// TwinCAT 3 PLC project Untitled1
// ProgramVersion: 3.1.4022.2
// libraries:
//   Tc2_Drive, * (Beckhoff Automation GmbH)
//   Tc2_MC2, * (Beckhoff Automation GmbH)
//   Tc2_MC2_Drive, * (Beckhoff Automation GmbH)
//   Tc2_Standard, * (Beckhoff Automation GmbH)
//   Tc2_System, * (Beckhoff Automation GmbH)
//   Tc2_Utilities, * (Beckhoff Automation GmbH)
//   Tc3_Module, * (Beckhoff Automation GmbH)
//   VisuSymbols,3.5.10.0,System
// project tree:
//   DUTs/ Alm_AlarmHistoryType.TcDUT, Alm_AlarmType.TcDUT, Alm_AlmMsg.TcDUT, Alm_EventClass.TcDUT, manualstep.TcDUT, ST_AlarmID.TcDUT, ST_AlarmString.TcDUT, ST_Setting.TcDUT, ST_States.TcDUT
//   / GlobalTextList.TcGTLO, PlcTask.TcTTO, Visualization Manager.TcVMO
//   GVLs/ _01_Global_Variables.TcGVL
//   POUs/ Axis_IO.TcPOU, Axis_PTP_CoE.TcPOU, FB_Home_ByLimit.TcPOU, MAIN.TcPOU, ServoDriver_DI.TcPOU
//   VISUs/Visualizations/PH/ PH_JOGLINE.TcVIS
//   VISUs/Visualizations/ Visualization.TcVIS
// real-time tasks:
//   TASK PlcTask: cycle T#10ms, priority 20, ADS port 350
// motion (NC):
//   TASK NC-Task 1 SAF: cycle T#2ms, priority 4, ADS port 501
//   TASK NC-Task 1 SVB: cycle T#10ms, priority 8, ADS port 511
//   AXIS Axis 1 (id 1)
//     Dynamic: Acceleration=13453.5, Deceleration=13453.5, Jerk=40360.6
//     Velo: RefSearch=89.69024, RefSync=89.69024, SlowManual=448.4512, FastManual=2690.7072, Fast=8969.024, Maximum=8969.02
//     OtherSettings: AllowMotionCmdToSlave=true
//     encoder EncType=8
//       EncPara: ScaleFactorNumerator=104.8576, ScaleFactorDenominator=1048576, MaxCount=#xffffffff
//     drive DrvType=9
//       DrvPara: MaxCount=#xffffffff, DriveControlDWord=#x00030100
//         Analog: VeloReferenz=9865.9264, VeloScale=1.02400649589962, ScaleFactorActTorque=0.1
//         TimeComp: TaskDelayCycles=1
//     controller CtrType=1
//       CtrPara: PriorControlFactor=1
//         Observer: BandWidth=20
//   AXIS Axis 2 (id 2)
//     Dynamic: Acceleration=13453.5, Deceleration=13453.5, Jerk=40360.6
//     Velo: RefSearch=89.69024, RefSync=89.69024, SlowManual=448.4512, FastManual=2690.7072, Fast=8969.024, Maximum=8969.02
//     OtherSettings: AllowMotionCmdToSlave=true
//     encoder EncType=8
//       EncPara: ScaleFactorNumerator=104.8576, ScaleFactorDenominator=1048576, MaxCount=#x0036ee7f
//     drive DrvType=9
//       DrvPara: MaxCount=#xffffffff, DriveControlDWord=#x00030100
//         Analog: VeloReferenz=9865.9264, VeloScale=6, ScaleFactorActTorque=0.1
//         TimeComp: TaskDelayCycles=1
//     controller CtrType=1
//       CtrPara: PriorControlFactor=1
//         Observer: BandWidth=20
// I/O:
//   DEVICE Device 1 (EtherCAT), AmsNetId 169.254.43.76.2.1
//     Term 1 (EK1200) [EK1200-5000 EtherCAT Power supply (2A E-Bus)]
//       Term 2 (EL1008) [EL1008 8Ch. Dig. Input 24V, 3ms]
//       Term 3 (EL2004) [EL2004 4Ch. Dig. Output 24V, 0.5A]
//       Term 4 (EL1259) [EL1259 8Ch. Dig Input 24V/8Ch. Dig. Output 24V with Multi-Time-Stamp]
//       Term 5 (EL1004) [EL1004 4Ch. Dig. Input 24V, 3ms]
//       Term 6 (EL2024) [EL2024 4Ch. Dig. Output 24V, 2A]
//       Term 7 (EL3204) [EL3204 4Ch. Ana. Input PT100 (RTD)]
//       Term 8 (EK1521) [EK1521 1 port EtherCAT junction (FX-MultiMode)]
//       Term 9 (EL6601) [EL6601 1 Port Switch (Ethernet, CoE)]
//       Term 10 (EL6731-0010) [EL6731-0010 PROFIBUS DP Slave]
//       Term 11 (EK1110) [EK1110 EtherCAT extension]
//     Term 12 (EK1100) [EK1100 EtherCAT Coupler (2A E-Bus)]
//       Term 13 (EL1004) [EL1004 4Ch. Dig. Input 24V, 3ms]
//       Term 14 (EL2004) [EL2004 4Ch. Dig. Output 24V, 0.5A]
//       Term 15 (EL6900) [EL6900, TwinSAFE PLC]
//       Term 16 (EL2904) [EL2904, 4 Ch. Safety Output 24V, 0.5A, TwinSAFE]
//         modules: Module 1 (FSOES), Module 2 (DO)
//       Term 17 (EL1904) [EL1904, 4 Ch. Safety Input 24V, TwinSAFE]
//         modules: Module 1 (FSOES)
//       Term 18 (EK1110) [EK1110 EtherCAT extension]
//     Drive 19 (AX5206-0000-0210) [AX5206-0000-0210 EtherCAT Drive (SoE, 2 Ch.)]
// variable links:
//   NC-Task 1 SAF/Axes/Axis 1 <-> Device 1 (EtherCAT)/Drive 19 (AX5206-0000-0210)
//     Drive/Inputs/In/nDataIn1 <-> AT 1/Following distance
//     Drive/Inputs/In/nDcOutputTime <-> InfoData/DcOutputShift
//     Drive/Inputs/In/nState1 <-> AT 1/Drive status word @bit 8
//     Drive/Inputs/In/nState2 <-> AT 1/Drive status word
//     Drive/Inputs/In/nState4 @bit 1 <-> WcState/InputToggle
//     Drive/Inputs/In/nState4 <-> WcState/WcState
//     Drive/Outputs/Out/nCtrl1 <-> MDT 1/Master control word @bit 8
//     Drive/Outputs/Out/nDataOut1 <-> MDT 1/Position command value
//     Enc/Inputs/In/nDataIn1 <-> AT 1/Position feedback 1 value
//     Enc/Inputs/In/nDcInputTime <-> InfoData/DcInputShift
//     Enc/Inputs/In/nState4 @bit 1 <-> WcState/InputToggle
//     Enc/Inputs/In/nState4 <-> WcState/WcState
//   NC-Task 1 SAF/Axes/Axis 2 <-> Device 1 (EtherCAT)/Drive 19 (AX5206-0000-0210)
//     Drive/Inputs/In/nDataIn1 <-> AT 2/Following distance
//     Drive/Inputs/In/nDcOutputTime <-> InfoData/DcOutputShift
//     Drive/Inputs/In/nState1 <-> AT 2/Drive status word @bit 8
//     Drive/Inputs/In/nState2 <-> AT 2/Drive status word
//     Drive/Inputs/In/nState4 @bit 1 <-> WcState/InputToggle
//     Drive/Inputs/In/nState4 <-> WcState/WcState
//     Drive/Outputs/Out/nCtrl1 <-> MDT 2/Master control word @bit 8
//     Drive/Outputs/Out/nDataOut1 <-> MDT 2/Position command value
//     Enc/Inputs/In/nDataIn1 <-> AT 2/Position feedback 1 value
//     Enc/Inputs/In/nDcInputTime <-> InfoData/DcInputShift
//     Enc/Inputs/In/nState4 @bit 1 <-> WcState/InputToggle
//     Enc/Inputs/In/nState4 <-> WcState/WcState
//   Untitled1/Untitled1 Instance <-> Device 1 (EtherCAT)/Drive 19 (AX5206-0000-0210)
//     PlcTask Inputs/MAIN.axis1.IO.DriverDI.ErrorCode <-> AT 1/Diagnostic number
//   Untitled1/Untitled1 Instance <-> Device 1 (EtherCAT)/Term 1 (EK1200)/Term 2 (EL1008)
//     PlcTask Inputs/MAIN.axis1.IO.DriverDI.EL1008 <-> Channel 1/Input
//     PlcTask Inputs/MAIN.axis1.IO.DriverDI.EL1008 @bit 1 <-> Channel 2/Input
//     PlcTask Inputs/MAIN.axis1.IO.DriverDI.EL1008 @bit 3 <-> Channel 4/Input
//     PlcTask Inputs/MAIN.axis1.IO.DriverDI.EL1008 @bit 4 <-> Channel 5/Input
//     PlcTask Inputs/MAIN.axis1.IO.DriverDI.EL1008 @bit 5 <-> Channel 6/Input
//     PlcTask Inputs/MAIN.axis1.IO.DriverDI.EL1008 @bit 6 <-> Channel 7/Input
//     PlcTask Inputs/MAIN.axis1.IO.DriverDI.EL1008 @bit 7 <-> Channel 8/Input
//     PlcTask Inputs/MAIN.home_exe <-> Channel 3/Input
//   Untitled1/Untitled1 Instance <-> Device 1 (EtherCAT)/Term 1 (EK1200)/Term 5 (EL1004)
//     PlcTask Inputs/MAIN.axis1.IO.DriverDI.EL1004 <-> Channel 1/Input
//   Untitled1/Untitled1 Instance <-> NC-Task 1 SAF/Axes/Axis 1
//     PlcTask Inputs/MAIN.axis1.Ref.NcToPlc <-> Outputs/ToPlc
//     PlcTask Outputs/MAIN.axis1.Ref.PlcToNc <-> Inputs/FromPlc

CONFIGURATION Untitled1
    RESOURCE PLC ON TwinCAT3
        TASK PlcTask(INTERVAL := T#10ms, PRIORITY := 20);
        PROGRAM MAIN WITH PlcTask : MAIN;
    END_RESOURCE
END_CONFIGURATION

// ---- DUTs/Alm_AlarmHistoryType.TcDUT
TYPE Alm_AlarmHistoryType :
STRUCT
  	EventMessage:            	WSTRING;
	EventId:					INT;
   	EventTime:               	DT;
END_STRUCT
END_TYPE

// ---- DUTs/Alm_AlarmType.TcDUT
TYPE Alm_AlarmType :
STRUCT
      (*InPut*)
	EventId:					INT;
    EventMessage:			WSTRING;
    EventTime:                                 DT;
	EventActive:				BOOL;
	QuitRequired:				BOOL;
	QuitEvent:				BOOL;
	EventClass:				Alm_EventClass;
	AlarmMsg:				Alm_AlmMsg;
	AlarmlampOn:			BOOL;(*报警灯*)
	AutoRunOff:				BOOL;(*退出自动循环*)

	(* event actions OutPut	*)
	AlarmAction1:				BOOL;
	AlarmAction2:				BOOL;
	AlarmAction3:				BOOL;
	AlarmAction4:				BOOL;
	AlarmAction5:				BOOL;
	AlarmAction6:				BOOL;
	AlarmAction7:				BOOL;
	AlarmAction8:				BOOL;

       (*OutPut*)
	EventAlive:					BOOL;
    ShowlampOn:           		BOOL;
	InUse:                		BOOL;
END_STRUCT
END_TYPE;

// ---- DUTs/Alm_AlmMsg.TcDUT
TYPE Alm_AlmMsg :
STRUCT
	CN:		WSTRING:="中文";
	EN:		STRING:='En';	
END_STRUCT
END_TYPE

// ---- DUTs/Alm_EventClass.TcDUT
TYPE Alm_EventClass :
(
    NoAlarm                  :=0,(*无警报*)
    Message_1      :=1,(*信息*)
    Event_2            :=2,(*事件*)
    non_3                        :=3,(*暂无*)
    non_4                       :=4,(*暂无*)
    non_5                         :=5,(*暂无*)
    Alarm_6          :=6,(*不停机警报*)
    Stop_7                :=7(*停机警报*)
);
END_TYPE

// ---- DUTs/manualstep.TcDUT

TYPE manualstep :
(
	moveoff:=0,
    jogB,
	jogF,
	homing ,
	MoveRel,
	MoveABS,
	MoveVel,
	stop
);
END_TYPE

// ---- DUTs/ST_AlarmID.TcDUT
TYPE ST_AlarmID :
(*报警的id号，swen*)
STRUCT
	(*系统*)
	EtherCATBusErr:					INT:=1;(*EtherCAT总线错误*)
	SystemLoading:					INT:=2;(*系统启动中*)
	EmergentStop:					INT:=3;(*急停按钮*)
	ProductChangeNeedSave:			INT:=4;
	ProductLoadingNoPowerOff:		INT:=5;
	AirPressLow:					INT:=6;(*气压低!*)
	Prushing:						INT:=7;(*暂停中*)
	NeedHoming:						INT:=8;(*开机前请先找原点*)
	IsHoming:						INT:=9;(*正在找原点*)
	AutoStoping:					INT:=10;(*自动停机中*)
	AutoStopImediery:				INT:=11;(*马上停机中*)
	AutoRuning:						INT:=12;(*设备运行中*)
	ComErrorVS:						INT:=13;(*视觉控制器通讯异常*)
	ServoError:						INT:=14;(*伺服出错*)
	ServoHwError:					INT:=15;(*伺服驱动器报错，硬件报错*)
	ServoLimit:						INT:=16;(*伺服驱动器限位到*)
	CycleTimeOut:					INT:=17;(*循环时间超时*)
	ModbusRtuError:					INT:=18;(*ModbusRtu总线错误*)
	RobotError1:					INT:=19;(*机器人错误*)
	RobotError2:					INT:=20;(*机器人错误*)
	StepServoError:					INT:=21;(*步进驱动器报错*)
	RobotSN_Error:					INT:=22;(*机器人序列号异常*)

	(*程序逻辑*)
	ClampVacuum:					INT:=26;(*机器人1真空吸取失败*)








	(*序列号*)
	Machime_SoftHwDif:				INT:=50;(*软硬件不匹配*)
	Machime_Alarm_NeedKey:			INT:=51;(*系统即将进入维护模式*)
	Machime_Stop_NeedKey:			INT:=52;(*系统已经进入维护模式*)

END_STRUCT
END_TYPE

// ---- DUTs/ST_AlarmString.TcDUT
TYPE ST_AlarmString :
STRUCT
	chinese:		STRING:='CN';
	english:		STRING:='EN';
END_STRUCT
END_TYPE

// ---- DUTs/ST_Setting.TcDUT
TYPE ST_Setting :
STRUCT
	(*系统*)
	gcSimulationMode:		BOOL;
	JogVelocity:			REAL:=20;
	AutoVelocity:			REAL:=500;(*皮带的速度*)
	ClampVelocity:			REAL:=2000;(*机械手的速度*)

	tCutTime:				REAL:=0.5;(*剪断时间*)

	ZPickUpHeight:			REAL:=200;(*抓起来的高度*)
	XPlacePos:				REAL:=450;(*抓过去的X距离*)
	YPlacePos:				REAL:=330;(*抓过去的Y距离*)
	ZPlacePos:				REAL:=-650;(*放到地板的高度*)
	Box_Longth:				REAL:=215;(*箱子长*)
	Box_Width:				REAL:=190;(*箱子宽*)
	Box_Height:				REAL:=198;(*箱子高*)

END_STRUCT
END_TYPE

// ---- DUTs/ST_States.TcDUT
TYPE ST_States :
STRUCT
	ManualModeIsActive:				BOOL;(*手动模式*)
	AutoModeIsActive:				BOOL;(*自动模式*)
	MachineRunInCycle:				BOOL;(*自动运行中*)
	GoPauseState:					BOOL;(*请求暂停记忆*)
	AutoStoping:					BOOL;(*自动停机中*)
	ResetAlarm:						BOOL;(*报警复位*)
	GoHome:							BOOL;(*请求找原点*)


	(*电机*)
	HomeDone:						BOOL;(*原点完成*)
	Motor_PowerOn:				BOOL;(*上电完成*)
	Motor_HomeDone:				BOOL;(*原点完成*)
	Motor_SwError:				BOOL;(*电机NC软件出错*)
	Motor_SwErrId:				UDINT;
	Motor_Limit:				BOOL;(*电机限位*)
	Motor_HwError:				BOOL;(*电机硬件出错*)

	Hmi_btHome:						BOOL;(*画面按钮*)(*回原点*)
	Hmi_btAutoRun:					BOOL;(*画面按钮*)(*开始*)
	Hmi_btAutoStop:					BOOL;(*画面按钮*)(*停止*)
	Hmi_btPause:					BOOL;(*画面按钮*)(*暂停*)


	(*状态*)
	ConvCanRun:						BOOL:=TRUE;(*传送带启动允许*)

	ActBoxId:						INT;(*当前进箱子的ID号*)


END_STRUCT
END_TYPE

// ---- GVLs/_01_Global_Variables.TcGVL
{attribute 'Tc2GvlVarNames'}
VAR_GLOBAL
	DATA:						ST_States;	(*状态*)
END_VAR

// ---- POUs/MAIN.TcPOU
PROGRAM MAIN
VAR
	axis1: Axis_PTP_CoE;	
    home_exe AT%I*:BOOL;
    mstep:manualstep;
	AutoMode: BOOL;
END_VAR

axis1.sName:="X轴";
axis1.areset( );                                //刷新IO，读取轴状态、复位
axis1.aPower( );                                //使能

IF axis1.Ref.Status.ControlLoopClosed AND NOT AutoMode THEN      //判断使能成功，调用手动模式下点动指令
axis1.aManualJOG(Velo:=100 ,);
END_IF


IF home_exe THEN axis1.aHome(execute:=TRUE);  
	ELSE axis1.aHome(execute:=FALSE);
END_IF

IF automode THEN                              //自动模式下的指令使用
logic();
END_IF

ACTION logic:
CASE mstep OF 
	moveoff:
	   axis1.aStop(execute:=FALSE);
	   axis1.aMoveOff();
	jogB:
	   axis1.aJogB(execute:=TRUE,velo:=100); 
	jogF:
	   axis1.aJogF(execute:=TRUE,velo:=100); 
    homing:  
       axis1.aHome(execute:=TRUE);
       IF axis1.done THEN
	    mstep:=moveoff;
       END_IF
	MoveRel:
	   axis1.aMoverel(execute:=TRUE,Target:=100,velo:=100);
	   IF axis1.done THEN
	    mstep:=moveoff;
	   END_IF
	Moveabs:
	   axis1.aMoveabs(execute:=TRUE,Target:=100,velo:=100);
	   IF axis1.done THEN
	    mstep:=moveoff;
	   END_IF
	MoveVel:
	   axis1.aMoveVel(execute:=TRUE,velo:=100);
    stop:
	   axis1.aStop(execute:=TRUE);
END_CASE
END_ACTION

END_PROGRAM

// ---- POUs/Axis_PTP_CoE.TcPOU
FUNCTION_BLOCK Axis_PTP_CoE
VAR_INPUT
	Execute:				BOOL;
	bReset:					BOOL;
	Ref:					AXIS_REF;
	IO:						Axis_IO;
	mcJog:					MC_Jog;
	mcHome:					FB_Home_ByLimit;
	mcMoveAbsolute:			MC_MoveAbsolute;
	mcMoveRelative:			MC_MoveRelative;
	mcMoveVelocity:			MC_MoveVelocity;
	mcSoEReset:				FB_SoEReset;
	mcPower:				MC_Power;
	mcReset:				MC_Reset;
	mcStop:					MC_Stop;

	Target					:	LREAL;
	Velo					: 	LREAL;
	Jerk					:	LREAL := 0.0;
	Acc						:	LREAL := 0.0;
	Dec						:	LREAL := 0.0;

	sName:					WSTRING:="轴";
END_VAR
VAR
	Done:					BOOL;(*功能块执行完成状态*)
	Busy: 					BOOL;(*功能块正在执行状态*)
	Active:					BOOL;
	CommandAborted:			BOOL;
	Error:					BOOL;
	ErrorID:				UDINT;
END_VAR

;

ACTION aHome:
(*
TYPE MC_HomingMode :
(
	MC_DefaultHoming,		(* default homing as defined in the SystemManager encoder parameters *)
	MC_AbsSwitch, 		(* not implemented - Absolute Switch homing plus Limit switches *)
	MC_LimitSwitch, 		(* not implemented - Homing against Limit switches *)
	MC_RefPulse, 		(* not implemented - Homing using encoder Reference Pulse "Zero Mark" *)
	MC_Direct, 		(* Static Homing forcing position from user reference *)
	MC_Absolute, 		(* not implemented - Static Homing forcing position from absolute encoder *)
	MC_Block, 		(* not implemented - Homing against hardware parts blocking movement *)
	MC_ForceCalibration, 	(* set the calibration flag without performing any motion or changing the position *)
	MC_ResetCalibration  	(* resets the calibration flag without performing any motion or changing the position *)
);
END_TYPE

*)


mcHome(
	Execute:= 			Execute,
	Position:= 			,
	HomingMode:= 		,
	PosLimit:=			IO.snLimitP,
	NegLimit:=			IO.snLimitN,
	bCalibrationCam:= 	IO.snHome,
	Axis:= 				Ref,
	Done=>				Done,
	Busy=> 			Busy,
	Active=> 		Active,
	CommandAborted=> CommandAborted,
	Error=> 		Error,
	ErrorID=> 		ErrorID
	);
END_ACTION

ACTION aIO:
IO.DriverDI();(*调用axis_io*)

IO.snLimitP	:=IO.DriverDI.bLimitSenser_P;
IO.snLimitN	:=IO.DriverDI.bLimitSenser_N;
IO.snHome	:=IO.DriverDI.bHomeSenser;


IF IO.snLimitP
OR IO.snLimitN THEN(*极限*)
	DATA.Motor_Limit:=TRUE;
END_IF

IF IO.DriverDI.bHwError THEN(*×硬件故障*)
	DATA.Motor_HwError:=TRUE;
END_IF

IF Ref.Status.Error THEN(*NC的故障状态*)
	DATA.Motor_SwError:=TRUE;
	DATA.Motor_SwErrId:=Ref.Status.ErrorID;
	
END_IF
END_ACTION

ACTION aJogB:
mcJog(
	JogForward:= 	FALSE,
	JogBackwards:= 	Execute,
	Mode:= 			MC_JOGMODE_CONTINOUS,
	Position:= 		,
	Velocity:= 		Velo,
	Acceleration:= 	Acc,
	Deceleration:= 	Dec,
	Jerk:= 			Jerk,
	Axis:= 			Ref,
	Busy=> 			Busy,
	Active=> 		Active,
	CommandAborted=> CommandAborted,
	Error=> 		Error,
	ErrorID=> 		ErrorID
	);
END_ACTION

ACTION aJogF:
mcJog(
	JogForward:= 	Execute,
	JogBackwards:= 	FALSE,
	Mode:= 			MC_JOGMODE_CONTINOUS,
	Position:= 		,
	Velocity:= 		Velo,
	Acceleration:= 	Acc,
	Deceleration:= 	Dec,
	Jerk:= 			Jerk,
	Axis:= 			Ref,
	Busy=> 			Busy,
	Active=> 		Active,
	CommandAborted=> CommandAborted,
	Error=> 		Error,
	ErrorID=> 		ErrorID
	);
END_ACTION

ACTION aManualJOG:
(*
TYPE E_JogMode :
(
	MC_JOGMODE_STANDARD_SLOW, (* motion with standard jog parameters for slow motion *)
	MC_JOGMODE_STANDARD_FAST, (* motion with standard jog parameters for fast motion *)
	MC_JOGMODE_CONTINOUS,     (* axis moves as long as the jog button is pressed using parameterized dynamics *)
	MC_JOGMODE_INCHING,       (* axis moves for a certain relative distance *)
	MC_JOGMODE_INCHING_MODULO (* axis moves for a certain relative distance - stop position is rounded to the distance value *)
);
END_TYPE

*)

mcJog(
	JogForward:= 	IO.btManualJogF,
	JogBackwards:= 	IO.btManualJogB,
	Mode:= 			MC_JOGMODE_CONTINOUS,
	Position:= 		,
	Velocity:= 		Velo,
	Acceleration:= 	Acc,
	Deceleration:= 	Dec,
	Jerk:= 			Jerk,
	Axis:= 			Ref,
	Busy=> 			Busy,
	Active=> 		Active,
	CommandAborted=> CommandAborted,
	Error=> 		Error,
	ErrorID=> 		ErrorID
	);
END_ACTION

ACTION aMoveAbs:
mcMoveAbsolute(
	Execute:= 		Execute,
	Position:= 		Target,
	Velocity:= 		Velo,
	Acceleration:= 	Acc,
	Deceleration:= 	Dec,
	Jerk:= 			Jerk,
	Axis:= 			Ref,
	Done=> 			Done,
	Busy=> 			Busy,
	Active=> 		Active,
	CommandAborted=> CommandAborted,
	Error=> 		Error,
	ErrorID=> 		ErrorID
	);
END_ACTION

ACTION aMoveOff:
(*触发条件复位*)
mcHome(
	Execute:= 		FALSE,
	Axis:= 			Ref,
	);

mcJog(
	JogForward:= 	FALSE,
	JogBackwards:= 	FALSE,
	Axis:= 			Ref,
	);

mcMoveAbsolute(
	Execute:= 		FALSE,
	Axis:= 			Ref,
	);

mcMoveRelative(
	Execute:= 		FALSE,
	Axis:= 			Ref,
	);

mcMoveVelocity(
	Execute:= 		FALSE,
	Axis:= 			Ref,
	);

Done:=FALSE;
Busy:=FALSE;
Active:=FALSE;
CommandAborted:=FALSE;
Error:=FALSE;
END_ACTION

ACTION aMoveRel:
mcMoveRelative(
	Execute:= 		Execute,
	Distance:= 		Target,
	Velocity:= 		Velo,
	Acceleration:= 	Acc,
	Deceleration:= 	Dec,
	Jerk:= 			Jerk,
	Axis:= 			Ref,
	Done=> 			Done,
	Busy=> 			Busy,
	Active=> 		Active,
	CommandAborted=> CommandAborted,
	Error=> 		Error,
	ErrorID=> 		ErrorID
	);
END_ACTION

ACTION aMoveVel:
mcMoveVelocity(
	Execute:= 		Execute,
	Direction:= 	,
	Velocity:= 		Velo,
	Acceleration:= 	Acc,
	Deceleration:= 	Dec,
	Jerk:= 			Jerk,
	Axis:= 			Ref,
	InVelocity=> 	Done,
	Busy=> 			Busy,
	Active=> 		Active,
	CommandAborted=> CommandAborted,
	Error=> 		Error,
	ErrorID=> 		ErrorID );
END_ACTION

ACTION aPower:
mcPower(
	Enable:= 			TRUE,
	Enable_Positive:= true	,
	Enable_Negative:=true 	,
	Override:= 		,
	BufferMode:= 	,
	Axis:= 			Ref,
	Status=> 		,
	Busy=> 			Busy,
	Active=> 		Active,
	Error=> 		Error,
	ErrorID=> 		ErrorID
	);
END_ACTION

ACTION aReset:
aIO();(*硬件IO刷新*)
Ref.ReadStatus();(*轴状态字刷新*)



(*NC复位*)
mcReset(
	Execute:= 	(bReset OR DATA.ResetAlarm)
				AND Ref.Status.Error,
	Axis:= 		Ref,
	);
(*AX5000驱动器复位*)
mcSoeReset(
	Execute:= 	(bReset OR DATA.ResetAlarm)
				AND Ref.Status.Error,
	Axis:= 		Ref,
	);


(*遇极限后禁止往极限方向运行*)
mcPower(
	Enable:= 			,
	Enable_Positive:= 	NOT IO.snLimitP
						
						AND mcPower.Enable,
	Enable_Negative:= 	NOT IO.snLimitN
					
						AND mcPower.Enable,
	Override:= 		,
	Axis:= 			Ref,

	);
END_ACTION

ACTION aStop:
aMoveOff(); (*触发条件复位*)
 
mcStop(
	Execute:= 		Execute,
	Deceleration:= 	Dec,
	Jerk:= 			Jerk,
	Options:= 		,
	Axis:= 			Ref,
	Done=> 			Done,
	Busy=> 			Busy,
	Active=> 		Active,
	CommandAborted=> CommandAborted,
	Error=> 		Error,
	ErrorID=> 		ErrorID
	);
END_ACTION

END_FUNCTION_BLOCK

// ---- POUs/Axis_IO.TcPOU
FUNCTION_BLOCK Axis_IO
VAR_INPUT
	snHome:			BOOL;(*原点*)
	snLimitP:		BOOL;(*正限*)
	snLimitN:		BOOL;(*负限*)
	btManualJogF:	BOOL;(*点动按钮正*)
	btManualJogB:	BOOL;(*点动按钮负*)
	DriverDI:		ServoDriver_DI;(*伺服驱动器的输入*)
END_VAR

;

END_FUNCTION_BLOCK

// ---- POUs/ServoDriver_DI.TcPOU
FUNCTION_BLOCK ServoDriver_DI(*伺服驱动器的数字量输入*)
VAR_INPUT

END_VAR
VAR_OUTPUT
END_VAR
VAR
	di_UDint AT%I*:			UDINT;(*数字量*)
	di_Uint AT%I*:			UINT;(*数字量*)
	ErrorCode AT%I*:		UDINT;(*伺服硬件错误号*)
	EL1008 AT%I*:           BYTE;
	EL1004 AT%I*:           BOOL;

	bHomeSenser:			BOOL;(*原点信号*)
	bLimitSenser_P:			BOOL;(*正向限位*)
	bLimitSenser_N:			BOOL;(*负向限位*)
	bHwError:					BOOL;(*硬件报警*)
END_VAR




	bHomeSenser 	:= di_UDint.2 OR di_Uint.2OR EL1004;	(*home=2, Plimit=1,Nlimit=0*)
	bLimitSenser_P 	:= di_UDint.1 OR di_Uint.4OR EL1008.0;
	bLimitSenser_N 	:= di_UDint.0 OR di_Uint.5OR EL1008.1;

IF errorcode=16#D012 OR errorcode=16#D013 THEN
	 bHwError			:= FALSE;
ELSE bHwError			:= TRUE; 
END_IF                                                       (* ErrorCode<>0;*)

END_FUNCTION_BLOCK

// ---- POUs/FB_Home_ByLimit.TcPOU
FUNCTION_BLOCK FB_Home_ByLimit
(*========================================
轴在任意位置回零功能块，无需考虑回零方向问题
默认回零方向：先负方向找原点,如果碰到负极限则改为正方向找原点

 By Swen & Richel	2017/2/8
==========================================*)
VAR_IN_OUT
	Axis				:	AXIS_REF;	(* B *)
END_VAR
VAR_INPUT
	Execute			:	BOOL;	(* B *)
	PosLimit		:BOOL;			(*正极限位信号*)
	NegLimit		:BOOL;			(*负极限位信号*)
	Position		:	LREAL			(* B *) := DEFAULT_HOME_POSITION;
	HomeingVelo		:LREAL	:=20;
	HomingMode		: 	MC_HomingMode;	(* V *)
	BufferMode		:	MC_BufferMode;		(* E *)
	Options			: 	ST_HomingOptions;	(* V *)	(* Beckhoff proprietary input *)
	bCalibrationCam 	: 	BOOL;	(* V *)	(* Beckhoff proprietary input *)


END_VAR
VAR_OUTPUT
	Done			:	BOOL;	(* B *)
	Busy			: 	BOOL;	(* E *)
	Active			: 	BOOL;	(* E *)
	CommandAborted	:	BOOL;	(* E *)
	Error			:	BOOL;	(* B *)
	ErrorID			:	UDINT;	(* E *)
END_VAR
VAR
	mcJog			:MC_Jog;
	mcHome			:MC_Home;
	HomeStep: INT;
END_VAR

IF  NOT Execute THEN
	mcJog.JogForward		:=FALSE;
	mcJog.JogBackwards		:=FALSE;
	mcHome.Execute			:=FALSE;
	done					:=FALSE;
	busy					:=FALSE;
	Error					:=FALSE;
	HomeStep				:=0;

END_IF


CASE HomeStep OF

0:
	busy	:=FALSE;
	Done	:=FALSE;
	IF 	Execute AND NOT Error  THEN

		IF	HomingMode  =MC_DefaultHoming  THEN  		 (*回零模式判断*)
			HomeStep	:=100;
		ELSE
			HomeStep	:=400;
		END_IF
		busy		:=TRUE;
		ErrorID		:=0;
	END_IF

100:
	mcJog.JogForward		:=FALSE;
	mcJog.JogBackwards		:=TRUE;		 (*先向负限位方向运动*)
	IF	NegLimit THEN
		mcJog.JogBackwards		:=FALSE;

		HomeStep	:=200;
	ELSIF  bCalibrationCam THEN
		mcJog.JogBackwards		:=FALSE;
		IF Axis.Status.NotMoving THEN
			HomeStep	:=400;
		END_IF
	ELSIF mcJog.Error THEN
			HomeStep	:=1000;

	END_IF

200:
	mcJog.JogBackwards		:=FALSE;
	mcJog.JogForward		:=TRUE;		(*向正限位方向运动*)

	IF	bCalibrationCam THEN
		HomeStep	:=300;
	ELSIF PosLimit THEN(*出错碰限位*)
		mcJog.JogForward		:=FALSE;
		HomeStep	:=1000;
	END_IF

300:

	mcJog.JogForward		:=FALSE;
	IF Axis.Status.NotMoving THEN
		HomeStep	:=400;
	END_IF


400:   (*调用回零功能块*)

	mcHome.Execute	:=TRUE;
	IF mcHome.Done AND AXIS.Status.Homed THEN
		done			:=TRUE;
		HomeStep	:=500;
	ELSIF AXIS.Status.Error THEN

		HomeStep	:=1000;
	END_IF

500:
	mcHome.Execute	:=FALSE;
	HomeStep		:=555;(*退出等待Execute下降沿*)

1000:
	Error			:=TRUE;
	IF	mcHome.ErrorID <> 0 THEN
		ErrorID			:=mcHome.ErrorID;
	ELSIF  mcJog.ErrorID <> 0 THEN
		ErrorID			:=mcJog.ErrorID;
	END_IF

	HomeStep		:=0;

END_CASE


Call_FB();

ACTION Call_FB:
mcJog
	(
	Velocity:=	HomeingVelo ,
	Mode:=		MC_JOGMODE_CONTINOUS ,
	Axis:=		Axis ,
	);

mcHome
	(
	Execute:= ,
	Position:=			Position ,
	HomingMode:= 		HomingMode,
	BufferMode:= 		BufferMode,
	Options:=			Options ,
	bCalibrationCam:=	bCalibrationCam ,
	Axis:=				Axis ,
	);
END_ACTION

END_FUNCTION_BLOCK

// ---- GlobalTextList.TcGTLO
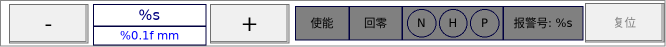
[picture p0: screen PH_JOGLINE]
VISUALIZATION PH_JOGLINE  // 666x47
VAR_IN_OUT
	m_Input_Name : Axis_PTP_CoE;
END_VAR
    RoundedRectangle (402,6 101x34)
    Rectangle (93,4 113x22), "%s", text variable: m_Input_Name.sName, text list: ''
    Button (210,4 79x39), "+"
        tap m_Input_Name.IO.btManualJogF
    Rectangle (93,26 113x19), "%0.1f mm", text variable: m_Input_Name.Ref.NcToPlc.ActPos, colour toggle: (m_Input_Name.Ref.Status.Moving) <> 0
    Button (9,4 79x39), "-"
        tap m_Input_Name.IO.btManualJogB
    RoundedRectangle (295,6 54x34), "使能", colour toggle: (m_Input_Name.Ref.Status.ControlLoopClosed) <> 0
    RoundedRectangle (349,6 53x34), "回零", colour toggle: (m_Input_Name.Ref.Status.Homed) <> 0
    RoundedRectangle (503,6 80x34), "报警号: %s", text variable: m_Input_Name.Ref.Status.ErrorID, colour toggle: (m_Input_Name.Ref.Status.Error) <> 0
    Ellipse (407,9 29x28), "N", colour toggle: (m_Input_Name.IO.snLimitN) <> 0
    Ellipse (470,9 29x28), "P", colour toggle: (m_Input_Name.IO.snLimitP) <> 0
    Ellipse (439,9 28x28), "H", colour toggle: (m_Input_Name.IO.snHome) <> 0
    Button (585,3 79x39), "复位"
        tap m_Input_Name.bReset
END_VISUALIZATION

// ---- VISUs/Visualizations/PH/PH_JOGLINE.TcVIS
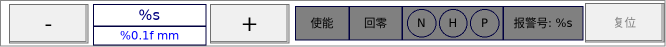
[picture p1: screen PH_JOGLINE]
VISUALIZATION PH_JOGLINE  // 666x47
VAR_IN_OUT
	m_Input_Name : Axis_PTP_CoE;
END_VAR
    RoundedRectangle (402,6 101x34)
    Rectangle (93,4 113x22), "%s", text variable: m_Input_Name.sName, text list: ''
    Button (210,4 79x39), "+"
        tap m_Input_Name.IO.btManualJogF
    Rectangle (93,26 113x19), "%0.1f mm", text variable: m_Input_Name.Ref.NcToPlc.ActPos, colour toggle: (m_Input_Name.Ref.Status.Moving) <> 0
    Button (9,4 79x39), "-"
        tap m_Input_Name.IO.btManualJogB
    RoundedRectangle (295,6 54x34), "使能", colour toggle: (m_Input_Name.Ref.Status.ControlLoopClosed) <> 0
    RoundedRectangle (349,6 53x34), "回零", colour toggle: (m_Input_Name.Ref.Status.Homed) <> 0
    RoundedRectangle (503,6 80x34), "报警号: %s", text variable: m_Input_Name.Ref.Status.ErrorID, colour toggle: (m_Input_Name.Ref.Status.Error) <> 0
    Ellipse (407,9 29x28), "N", colour toggle: (m_Input_Name.IO.snLimitN) <> 0
    Ellipse (470,9 29x28), "P", colour toggle: (m_Input_Name.IO.snLimitP) <> 0
    Ellipse (439,9 28x28), "H", colour toggle: (m_Input_Name.IO.snHome) <> 0
    Button (585,3 79x39), "复位"
        tap m_Input_Name.bReset
END_VISUALIZATION

// ---- VISUs/Visualizations/Visualization.TcVIS
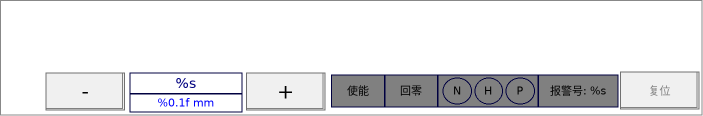
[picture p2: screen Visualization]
VISUALIZATION Visualization  // 703x116
    Frame (37,69 664x45)
        shows PH_JOGLINE(m_Input_Name := MAIN.axis1)
END_VISUALIZATION
